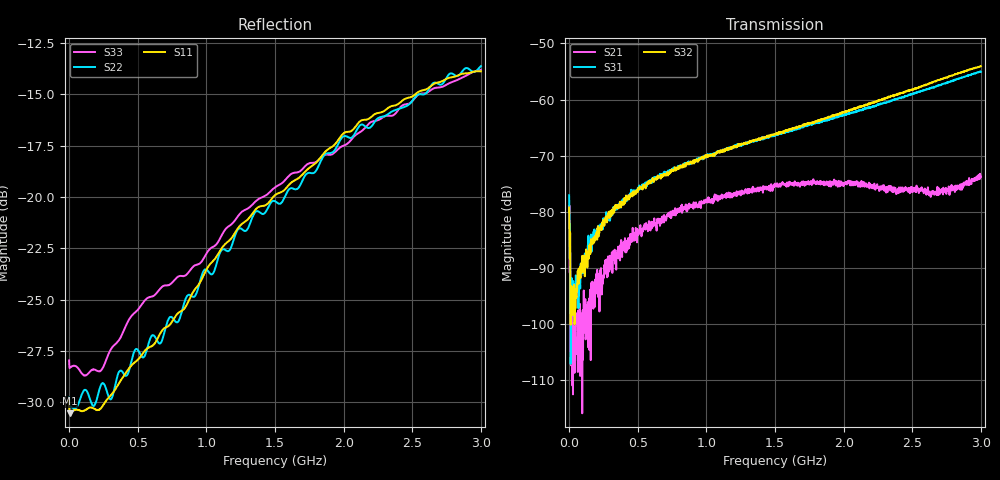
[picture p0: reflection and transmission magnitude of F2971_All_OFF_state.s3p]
! Frequency:  300kHz to 3GHz
! Package:  4mm x 4mm LQFN Plastic Package: 20 pin with exposed paddle.
!  Pin 1,2,4,5,6,7,9,10,11,12,14,15,18,19 = GND
!  Pin 3  = RF1  = Port 1
!  Pin 8  = RFC  = Port 3
!  Pin 13 = RF2  = Port 2
!  Pin 16 = C2
!  Pin 17 = C1
!  Pin 20 = VDD
!  E.P.  = GND
! State:  All OFF State
! Voltage:  VDD  = +3.0V
!  C1  = 0V (Logic LOW)
!  C2  = 0V (Logic LOW)
! Data:  The device was measured on the F2971 EVKit using a calibrated
!  network analyzer. The results below remove the PCB trace and
!  connector effects using the Automatic Fixture Removal software
!  from Keysight. Therfore, the reference plane for these results
!  are at the device's RF pin.
! Misc:
! Date:  2018-03-27  SJ
! Note:
!  Integrated Device Technology supplies this data as a sample of
!  measured data. Data was taken at 25 degrees C. Integrated Device
!  Technology reserves the right to change this data at anytime.
# hz S db R 75
! 3 Port Network Data from SP1.SP block
! freq  dbS11  angS11  dbS12  angS12  dbS13  angS13
!  dbS21  angS21
!  dbS22  angS22  dbS23  angS23
!  dbS31  angS31  dbS32  angS32
!  dbS33  angS33
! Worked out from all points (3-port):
!   1601 points, 30 kHz to 3 GHz, reference 75 ohm
!   strongest paths, dB at 30 kHz, 750 MHz, 1.5 GHz, 2.25 GHz, 3 GHz:
!     S32: -79.3, -72.6, -66.2, -60.3, -54.0
!     S31: -77.1, -72.6, -66.2, -61.0, -55.0
!     S21: -81.7, -80.3, -75.3, -75.8, -73.8
!   lowest |S11| = -30.5 dB at 5.655 MHz (marker M1), VSWR 1.06, Z = 70.7 + j0.06 ohm
!   |S11| at or under -10 dB: start of sweep to end of sweep
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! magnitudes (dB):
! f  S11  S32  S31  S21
! 30 kHz  -29.9  -79.3  -77.1  -81.7
! 5.655 MHz  -30.5  -88.5  -85.0  -90.9
! 16.9 MHz  -30.5  -97.5  -96.1  -104.8
! 225 MHz  -30.3  -82.9  -83.1  -91.7
! 305.7 MHz  -29.6  -80.2  -79.9  -88.8
! 714.4 MHz  -26.3  -73.2  -73.2  -80.5
! 1.5 GHz  -19.9  -66.2  -66.2  -75.3
! 2.027 GHz  -16.8  -62.1  -62.5  -74.8
! 2.683 GHz  -14.4  -56.6  -57.5  -75.6
! 3 GHz  -13.9  -54.0  -55.0  -73.8
